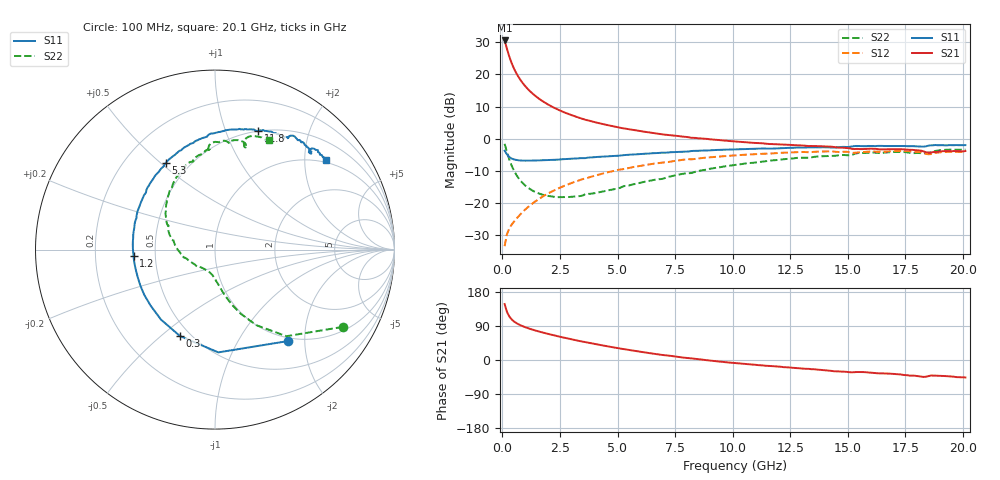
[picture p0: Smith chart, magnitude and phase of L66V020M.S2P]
!  Infineon Technologies AG
! BFR380L3 , PF131585-7, No.6, Th 09.10.01, soldered on pcb-board, measured with PP GSG850
!  Vce=6.0 V,  Ic=20.0 mA
! Common Emitter S-Parameters:  15. November 2001
#  GHz  S  MA  R  50
! f  S11  S21  S12  S22
! GHz  Mag  Ang  Mag  Ang  Mag  Ang  Mag  Ang
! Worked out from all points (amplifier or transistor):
!   201 points, 100 MHz to 20.1 GHz, reference 50 ohm
!   highest |S21| = 30.6 dB at 100 MHz (marker M1)
!   |S21| within 3 dB of that: start of sweep to 218.2 MHz
!   unconditionally stable (mu >= 1): 1.488 GHz to 4.371 GHz
!   at 3.4 GHz: K = 1.02, MAG = 8.7 dB, |S12| = -12.8 dB
!   at 10.1 GHz: K = 0.94, MSG = 2.2 dB, |S12| = -5.2 dB
!   at 20.1 GHz: K = 0.98, MSG = 0.1 dB, |S12| = -4.1 dB
!   S11 on the Smith chart (normalised r, x): 100 MHz: 0.94, -1.66; 300 MHz: 0.44, -0.58; 1.2 GHz: 0.37, -0.04; 5.3 GHz: 0.37, +0.52; 11.8 GHz: 0.50, +1.31; 20.1 GHz: 0.93, +2.52
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0.1  0.6511 -51.5  33.74 147.6  0.0213 65.1  0.8327 -31.1
0.2  0.573 -88.1  25.11 127.2  0.0326 57.2  0.6256 -50.5
0.3  0.5197 -112.1  19.09 115.3  0.04 54.4  0.4799 -61.3
0.4  0.4926 -127.7  15.15 107.5  0.04573 54.1  0.3851 -68.1
0.5  0.4755 -139.0  12.47 102.0  0.05101 55.2  0.3217 -72.9
0.6  0.4678 -147.6  10.56 97.9  0.05659 56.6  0.2776 -76.3
0.7  0.4616 -154.3  9.165 94.3  0.06186 57.9  0.2449 -79.2
0.8  0.4576 -159.6  8.078 91.3  0.06768 59.1  0.2204 -81.6
0.9  0.4556 -164.4  7.223 88.8  0.07352 60.0  0.2014 -83.7
1  0.4552 -168.3  6.539 86.4  0.07938 60.8  0.1865 -85.8
1.2  0.4556 -175.2  5.492 82.2  0.09142 61.9  0.1648 -89.7
1.6  0.4599 174.2  4.171 75.0  0.1165 62.9  0.1402 -97.2
2.1  0.4675 163.8  3.226 67.1  0.148 62.2  0.1273 -107.1
2.7  0.482 153.3  2.561 58.7  0.1854 60.1  0.1236 -119.7
3.5  0.4984 141.0  2.026 48.2  0.2357 56.2  0.131 -134.2
5.3  0.5564 119.4  1.441 28.5  0.3387 45.5  0.1838 -168.3
6.8  0.6003 104.2  1.191 14.5  0.4206 35.5  0.2346 168.6
10.1  0.6824 79.2  0.9054 -8.0  0.5497 14.1  0.3909 132.5
11.8  0.7041 70.0  0.8218 -16.4  0.5932 3.7  0.4616 116.2
13.5  0.7318 61.5  0.7694 -24.3  0.6242 -7.0  0.518 103.1
16.8  0.7707 48.8  0.6851 -35.9  0.6337 -23.4  0.6164 80.7
20.1  0.7943 39.0  0.6432 -46.1  0.6273 -37.4  0.6782 63.9
